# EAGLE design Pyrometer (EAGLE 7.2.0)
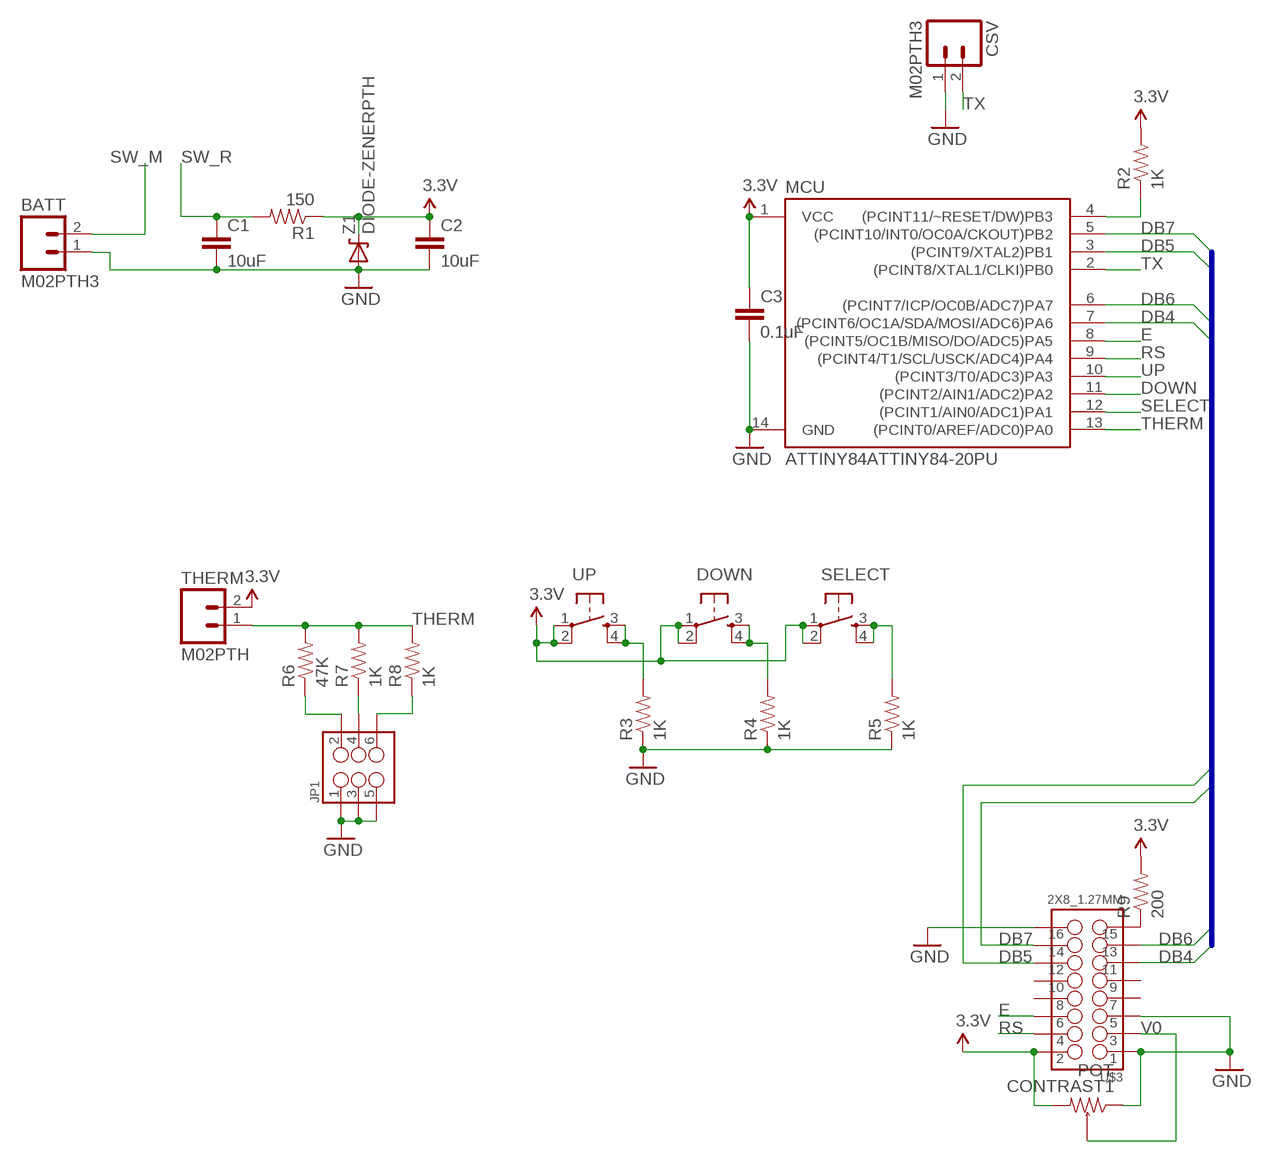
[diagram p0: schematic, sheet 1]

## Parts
BATT  M02PTH3  [1X02_LONGPADS]
C1  10uF  CAPEZ  [CAP-PTH-SMALLEZ]
C2  10uF  CAPEZ  [CAP-PTH-SMALLEZ]
C3  0.1uF  CAPEZ  [CAP-PTH-SMALLEZ]
CONTRAST1  POT  [POT]
CSV  M02PTH3  [1X02_LONGPADS]
DOWN  TAC_SWITCHPTH  [TACTILE-PTH]
JP1  M03X22X3_SILK_SM  [2X3]
MCU  ATTINY84ATTINY84-20PU  [DIL14]
R1  150  RESISTORPTH-1/4W  [AXIAL-0.4]
R2  1K  RESISTORPTH-1/4W  [AXIAL-0.4]
R3  1K  RESISTORPTH-1/4W  [AXIAL-0.4]
R4  1K  RESISTORPTH-1/4W  [AXIAL-0.4]
R5  1K  RESISTORPTH-1/4W  [AXIAL-0.4]
R6  47K  RESISTORPTH-1/4W  [AXIAL-0.4]
R7  1K  RESISTORPTH-1/4W  [AXIAL-0.4]
R8  1K  RESISTORPTH-1/4W  [AXIAL-0.4]
R9  200  RESISTORPTH-1/4W  [AXIAL-0.4]
SELECT  TAC_SWITCHPTH  [TACTILE-PTH]
THERM  M02PTH  [1X02]
U$3  2X8_1.27MM  [2X8_1.27MM]
UP  TAC_SWITCHPTH  [TACTILE-PTH]
Z1  DIODE-ZENERPTH  [DIODE-ZENER]

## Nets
3.3V: C2.1 C3.1 CONTRAST1.P$1 DOWN.1 DOWN.2 MCU.1(VCC) R1.P$1 R2.P$2 R9.P$2 SELECT.1 SELECT.2 THERM.2 U$3.P$2 UP.1 UP.2 Z1.P$1(C)
DB4: MCU.7((PCINT6/OC1A/SDA/MOSI/ADC6)PA6) U$3.P$11
DB5: MCU.3((PCINT9/XTAL2)PB1) U$3.P$12
DB6: MCU.6((PCINT7/ICP/OC0B/ADC7)PA7) U$3.P$13
DB7: MCU.5((PCINT10/INT0/OC0A/CKOUT)PB2) U$3.P$14
DOWN: DOWN.3 DOWN.4 MCU.11((PCINT2/AIN1/ADC2)PA2) R4.P$2
E: MCU.8((PCINT5/OC1B/MISO/DO/ADC5)PA5) U$3.P$6
GND: BATT.1 C1.2 C2.2 C3.2 CONTRAST1.P$3 CSV.1 JP1.1 JP1.3 JP1.5 MCU.14(GND) R3.P$1 R4.P$1 R5.P$1 U$3.P$1 U$3.P$5 U$3.P$16 Z1.P$2(A)
N$2: MCU.4((PCINT11/~RESET/DW)PB3) R2.P$1
N$3: JP1.4 R7.P$1
N$4: JP1.2 R6.P$1
N$5: JP1.6 R8.P$1
N$6: R9.P$1 U$3.P$15
RS: MCU.9((PCINT4/T1/SCL/USCK/ADC4)PA4) U$3.P$4
SELECT: MCU.12((PCINT1/AIN0/ADC1)PA1) R5.P$2 SELECT.3 SELECT.4
SW_M: BATT.2
SW_R: C1.1 R1.P$2
THERM: MCU.13((PCINT0/AREF/ADC0)PA0) R6.P$2 R7.P$2 R8.P$2 THERM.1
TX: CSV.2 MCU.2((PCINT8/XTAL1/CLKI)PB0)
UP: MCU.10((PCINT3/T0/ADC3)PA3) R3.P$2 UP.3 UP.4
V0: CONTRAST1.SWEEP U$3.P$3
Unconnected: U$3.P$7 U$3.P$8 U$3.P$9 U$3.P$10

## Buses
DB[4..7]

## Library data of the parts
BATT CSV THERM = SparkFun-Connectors:M02: Standard 2-pin 0.1" header. Use with
C1-C3 = SparkFun-Passives:CAP: Capacitor
CONTRAST1 = daniel:POT: 82PR10KLFTB Used in the mouser pyrometer project
DOWN SELECT UP = SparkFun-Electromechanical:TAC_SWITCH: Momentary Switch Button commonly used for reset or general input. Spark Fun Electronics SKU : COM-00097 SMT- SWCH-08247
JP1 = SparkFun-Connectors:M03X2: 2x3 .1" header. Shrouded, with keying- CONN-10681 SMT- CONN-11415 Pogo pins- HW-11044
MCU = SparkFun-DigitalIC:ATTINY84: Atmel 14-pin 2/4/8kB flash uC
R1-R9 = SparkFun-Resistors:RESISTOR: Resistor
U$3 = daniel:2X8_1.27MM
Z1 = SparkFun-DiscreteSemi:DIODE-ZENER: Zener Diode

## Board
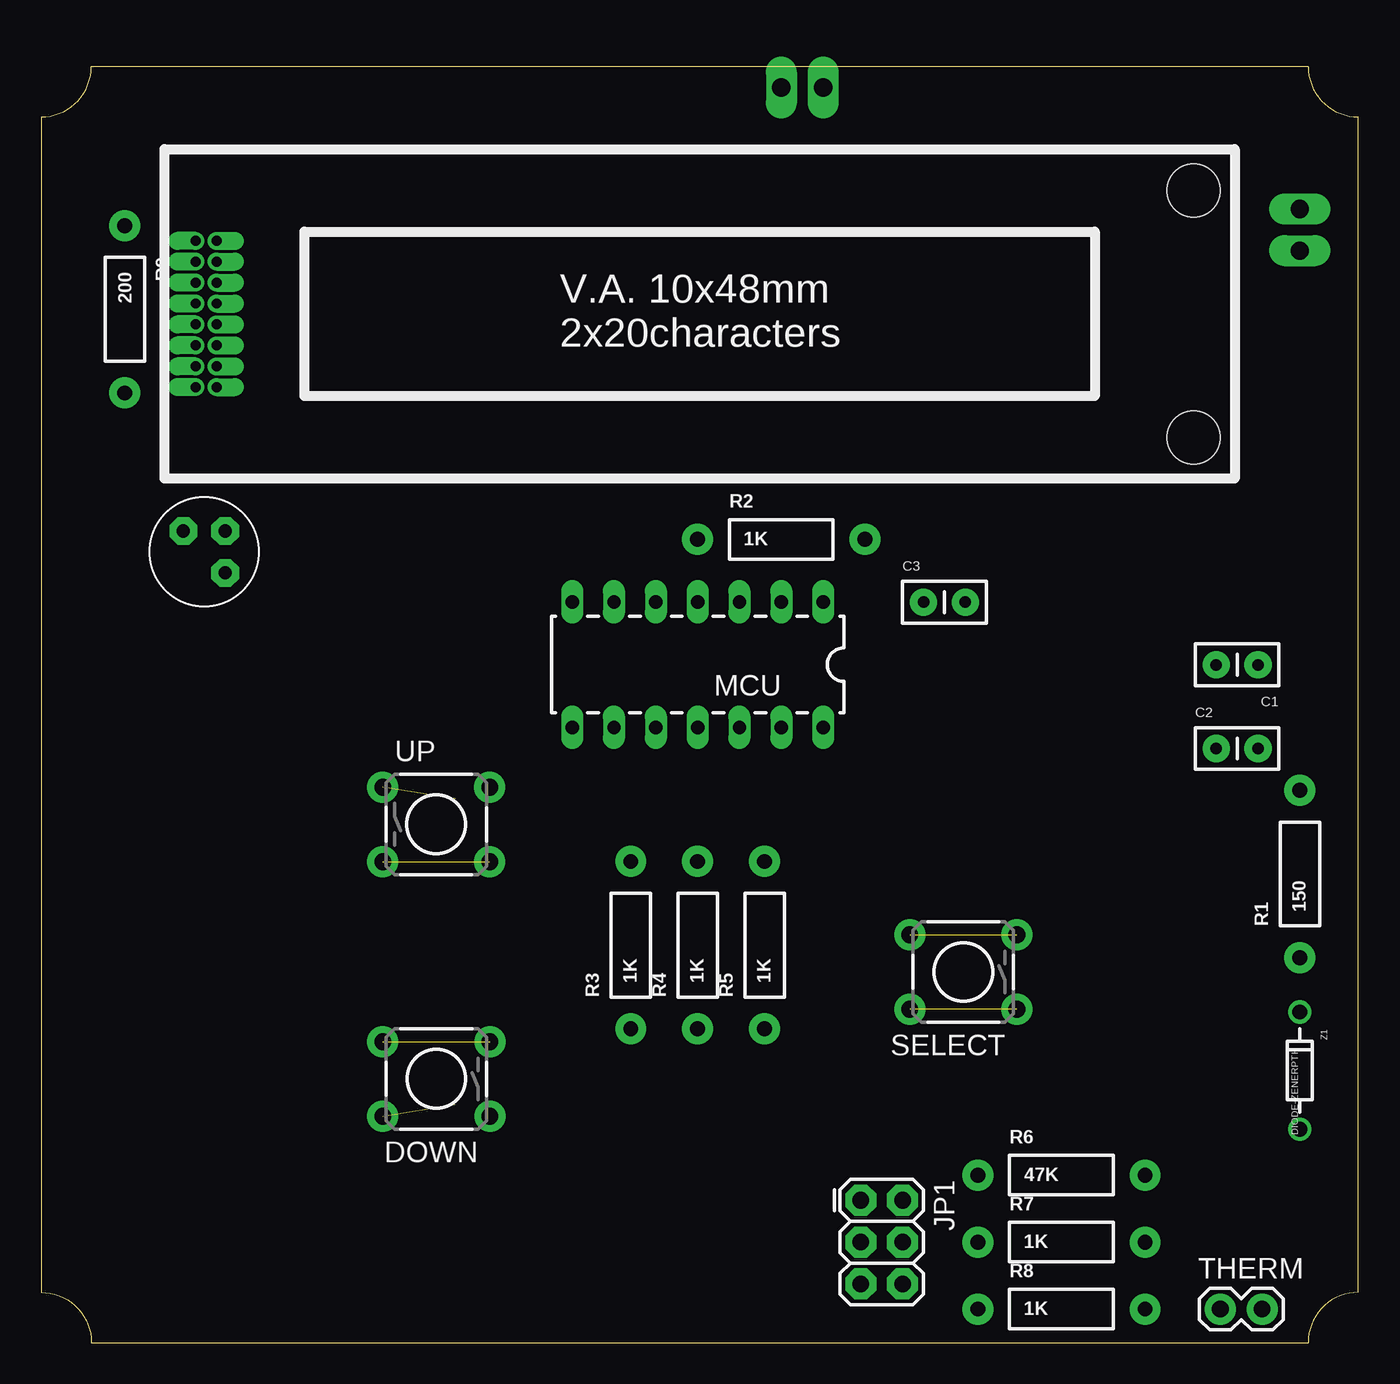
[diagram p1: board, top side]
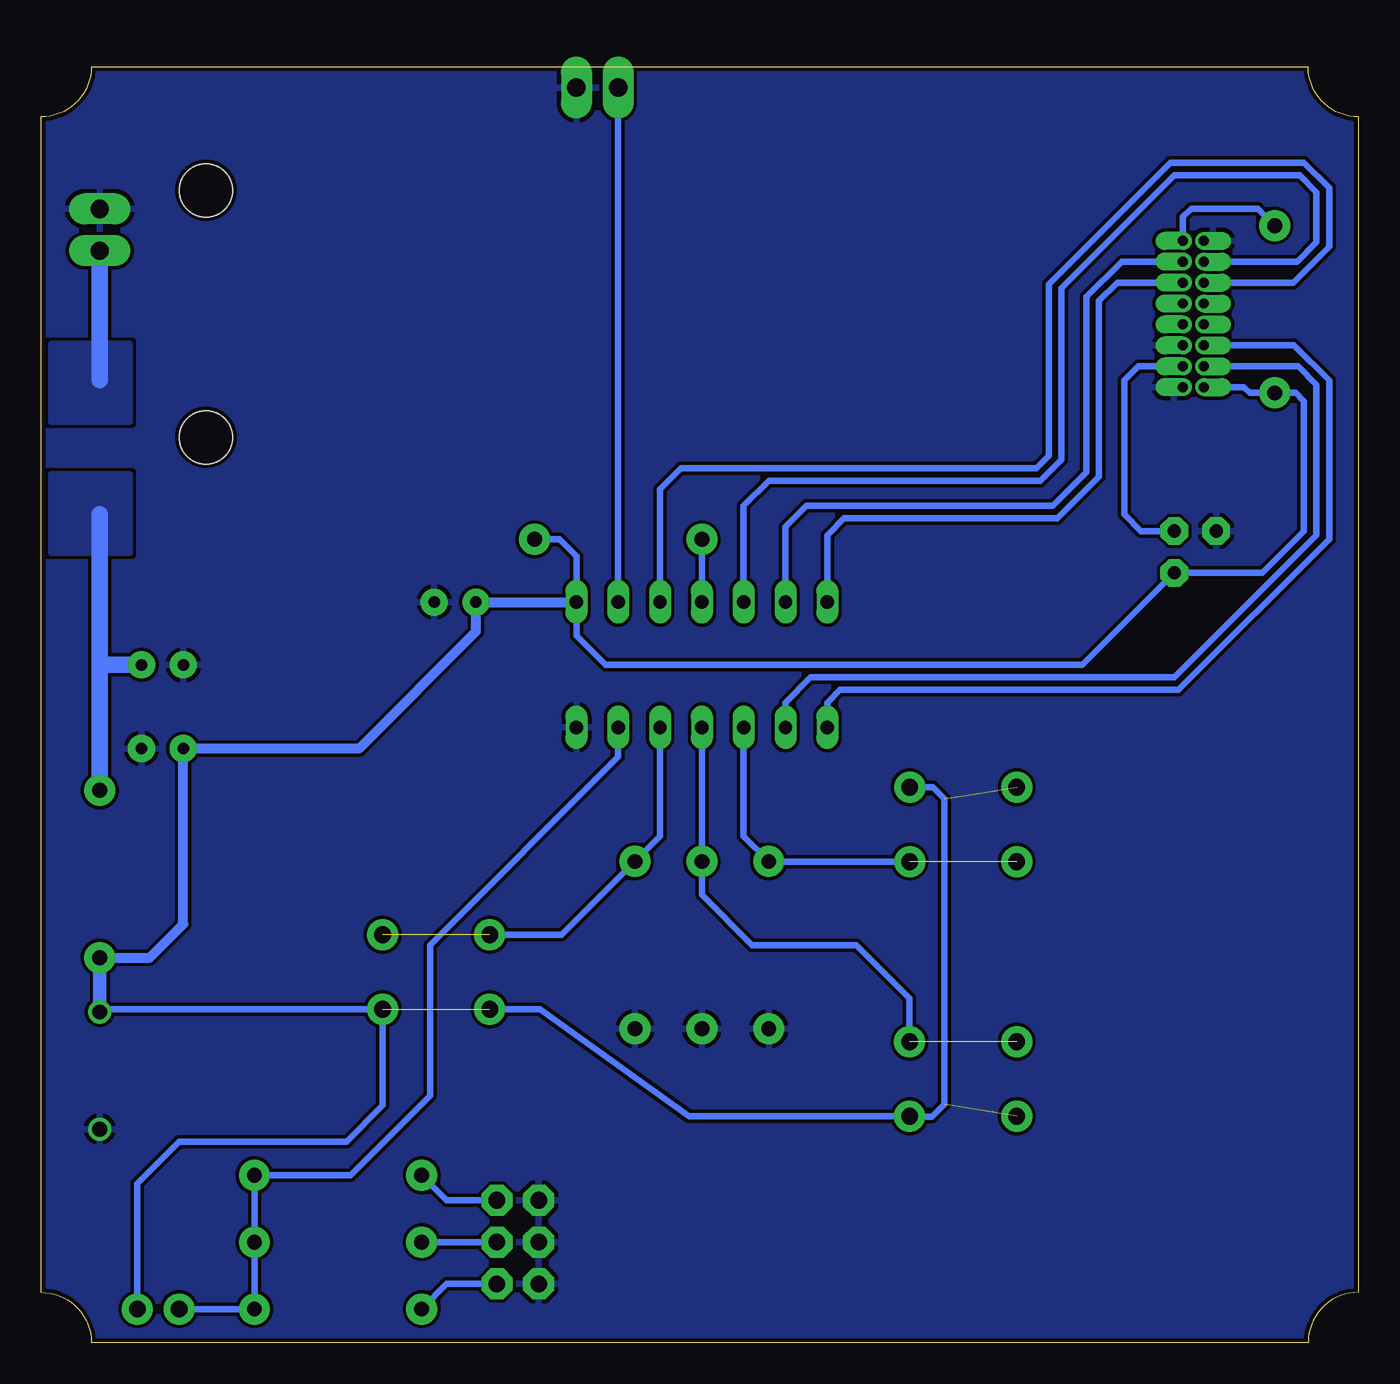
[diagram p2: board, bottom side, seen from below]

Size 80.01 x 77.47 mm. Coordinates in mm from the lower left corner, seen from the top.
Outline: 0.02,3.05 0,74.42 arc90 3.05,77.47 76.96,77.47 arc90 80.01,74.42 80.01,3.05 arc90 76.96,0 3.05,0 arc90 0,3.05
Copper layers (1*16): Top 0.035mm / dielectric 1.5mm / Bottom 0.035mm
Design rules "default *": minimum track width 10mil, minimum drill 24mil, track to track 8mil, track to pad 8mil, pad to pad 8mil, via to via 8mil, smd to smd 8mil, copper to edge 10mil, drill to drill 8mil, minimum pad ring 10mil, minimum via ring 8mil, stop-mask expansion 4mil, vias tented up to drill 0mil, thermal gap 10mil
Holes 3.2 mm at 70,69.96 70,54.96

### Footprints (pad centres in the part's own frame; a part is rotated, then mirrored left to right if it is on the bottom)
1X02_LONGPADS = drill 1.118 pad 1.88 long: 1 0,0; 2 2.54,0
CAP-PTH-SMALLEZ = drill 0.7 pad 1.651: 1 0,0; 2 2.54,0
POT = drill 0.8 pad 1.676 octagon: P$1 0,2.54; P$3 2.54,0; SWEEP 0,0
TACTILE-PTH = drill 1.016 pad 1.88: 1 -3.251,2.261; 2 3.251,2.261; 3 -3.251,-2.261; 4 3.251,-2.261
2X3 = drill 1.016 pad 1.88 octagon: 1 0,0; 2 0,2.54; 3 2.54,0; 4 2.54,2.54; 5 5.08,0; 6 5.08,2.54
DIL14 = drill 0.813 long: 1 -8.89,-3.81; 2 -6.35,-3.81; 3 -3.81,-3.81; 4 -1.27,-3.81; 5 1.27,-3.81; 6 3.81,-3.81; 7 6.35,-3.81; 8 6.35,3.81; 9 3.81,3.81; 10 1.27,3.81; 11 -1.27,3.81; 12 -3.81,3.81; 13 -6.35,3.81; 14 -8.89,3.81
AXIAL-0.4 = drill 0.9 pad 1.88: P$1 -5.08,0; P$2 5.08,0
1X02 = drill 1.016 pad 1.88: 1 0,0; 2 2.54,0
2X8_1.27MM = drill 0.6 pad 1.016 offset: P$1 0,0; P$2 -1.27,0; P$3 0,1.27; P$4 -1.27,1.27; P$5 0,2.54; P$6 -1.27,2.54; P$7 0,3.81; P$8 -1.27,3.81; P$9 0,5.08; P$10 -1.27,5.08; P$11 0,6.35; P$12 -1.27,6.35; P$13 0,7.62; P$14 -1.27,7.62; P$15 0,8.89; P$16 -1.27,8.89
DIODE-ZENER = drill 0.9: P$1 -3.556,0; P$2 3.556,0

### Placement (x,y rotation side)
BATT  76.45,68.83 270 top
C1  73.91,41.15 180 top
C2  71.37,36.07 0 top
C3  53.59,44.96 0 top
CONTRAST1  11.18,49.28 180 top
CSV  47.5,76.2 180 top
DOWN  24.01,16 180 top
JP1  49.78,8.64 270 top
MCU  38.61,41.16 180 top
R1  76.45,28.45 90 top
R2  44.96,48.77 0 top
R3  35.81,24.13 90 top
R4  39.88,24.13 90 top
R5  43.94,24.13 90 top
R6  61.98,10.16 0 top
R7  61.98,6.1 0 top
R8  61.98,2.03 0 top
R9  5.08,62.74 270 top
SELECT  56.01,22.5 180 top
THERM  71.63,2.03 0 top
U$3  10.65,58.01 0 top
UP  24,31.46 0 top
Z1  76.45,16.51 270 top

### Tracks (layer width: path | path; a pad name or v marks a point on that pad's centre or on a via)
3.3V  (3 unrouted)
  Bottom 0.406: U$3.P$2 6.96,58.01 6.6,57.66 R9.P$2 3.81,57.66 3.3,57.15 3.3,49.28 5.84,46.74 CONTRAST1.P$1 16.76,41.15 45.72,41.15 47.5,42.93 MCU.1 | UP.2 25.85,33.72 25.15,33.02 25.15,14.48 25.91,13.72 27.23,13.72 DOWN.1 40.67,13.74 49.7,20.24 SELECT.2 | MCU.1 47.5,47.75 48.51,48.77 R2.P$2 | 47.51,44.96 MCU.1 | THERM.2 74.17,9.65 71.63,12.19 61.47,12.19 59.27,14.39 SELECT.1 76.45,20.24 Z1.P$1
  Bottom 0.61: 47.51,44.96 C3.1 53.59,43.18 60.71,36.07 C2.1 71.37,25.4 73.41,23.37 R1.P$1
  Bottom 0.813: R1.P$1 Z1.P$1
DB4
  Bottom 0.406: MCU.7 32.26,49.02 31.24,50.04 18.29,50.04 15.75,52.58 15.75,63.25 14.63,64.36 U$3.P$11
DB5
  Bottom 0.406: MCU.3 42.42,51.82 41.15,53.09 19.56,53.09 18.8,53.85 18.8,64.26 11.43,71.63 3.3,71.63 1.78,70.1 1.78,66.55 3.97,64.36 U$3.P$12
DB6
  Bottom 0.406: MCU.6 34.8,49.53 33.53,50.8 18.54,50.8 16.51,52.83 16.51,63.5 14.38,65.63 U$3.P$13
DB7
  Bottom 0.406: MCU.5 37.34,50.8 35.81,52.32 19.3,52.32 18.03,53.59 18.03,64.01 11.18,70.87 3.56,70.87 2.54,69.85 2.54,66.8 3.71,65.63 U$3.P$14
DOWN  (1 unrouted)
  Bottom 0.406: MCU.11 R4.P$2 39.88,27.18 36.83,24.13 30.48,24.13 27.26,20.91 DOWN.3
E
  Bottom 0.406: U$3.P$6 3.91,60.55 1.78,58.42 1.78,48.77 10.92,39.62 31.5,39.62 32.26,38.86 MCU.8
GND
  pour Bottom (rank 2): 0,0 80.01,0 80.01,77.47 0,77.47
N$2
  Bottom 0.406: MCU.4 R2.P$1
N$3
  Bottom 0.406: JP1.4 R7.P$1
N$4
  Bottom 0.406: JP1.2 55.37,8.64 R6.P$1
N$5
  Bottom 0.406: JP1.6 55.37,3.56 R8.P$1
N$6
  Bottom 0.406: U$3.P$15 10.65,68.34 10.16,68.83 6.1,68.83 R9.P$1
RS
  Bottom 0.406: U$3.P$4 3.65,59.28 2.54,58.17 2.54,49.02 11.18,40.39 33.27,40.39 34.8,38.86 MCU.9
SELECT  (1 unrouted)
  Bottom 0.406: MCU.12 42.42,30.73 R5.P$2 48.39,24.76 SELECT.4
SW_M
  Bottom 1.016: BATT.2 76.45,58.42
  pour Bottom: 79.39,55.9 79.39,60.66 74.62,60.66 74.62,55.9
SW_R
  Bottom 1.016: 76.45,41.15 76.45,50.29 | C1.1 76.45,41.15 | R1.P$2 76.45,41.15
  pour Bottom: 79.39,52.72 74.62,52.72 74.62,47.96 79.39,47.96
THERM
  Bottom 0.406: THERM.1 R8.P$2 R7.P$2 R6.P$2 61.21,10.16 56.39,14.99 56.39,24.13 44.96,35.56 MCU.13
TX
  Bottom 0.406: CSV.2 MCU.2
UP  (1 unrouted)
  Bottom 0.406: UP.4 R3.P$2 37.34,30.73 MCU.10
V0
  Bottom 0.406: CONTRAST1.SWEEP 13.21,49.28 14.22,50.29 14.22,58.42 13.36,59.28 U$3.P$3

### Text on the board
tPlace: V.A. 10x48mm / 2x20characters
